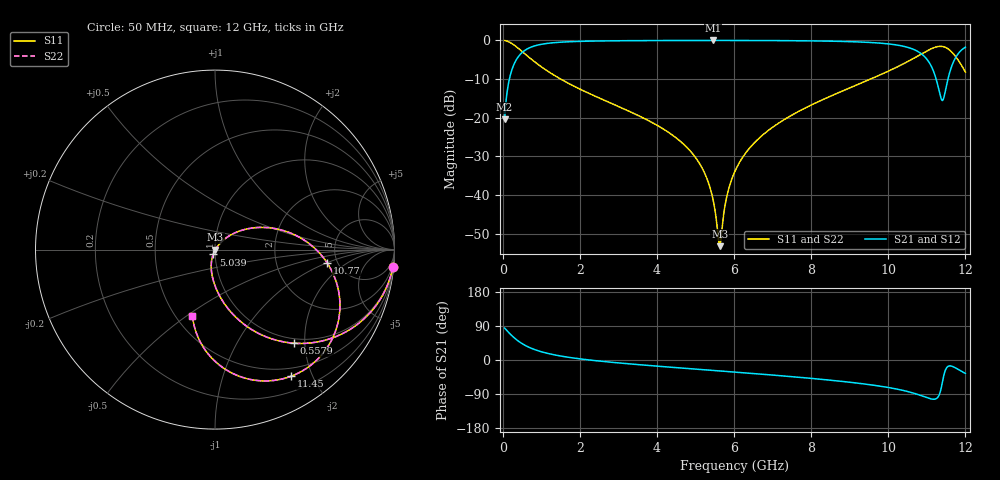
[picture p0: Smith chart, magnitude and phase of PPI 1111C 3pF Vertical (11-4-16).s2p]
# GHz S MA R 50
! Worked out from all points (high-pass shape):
!   1601 points, 50 MHz to 12 GHz, reference 50 ohm
!   highest |S21| = -0.02 dB at 5.457 GHz (marker M1); lowest = -20.4 dB at 50 MHz (marker M2)
!   |S21| within 3 dB of the highest: 518.8 MHz to 10.79 GHz (10.27 GHz wide, 182 % of centre); 11.85 GHz to end of sweep
!   lowest |S11| = -53.3 dB at 5.629 GHz (marker M3), VSWR 1.00, Z = 50.2 - j0.096 ohm
!   |S11| at or under -10 dB: 1.501 GHz to 9.544 GHz (8.043 GHz wide, 146 % of centre)
!   |S22| runs from -53.3 to 0.0 dB; largest |S21 - S12| = 0
!   S11 on the Smith chart (normalised r, x): 50 MHz: 1, -20; 557.9 MHz: 0.91, -1.77; 5.039 GHz: 0.98, -0.05; 10.77 GHz: 4.13, -0.99; 11.45 GHz: 0.39, -1.70; 12 GHz: 0.61, -0.52
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0.05  0.9954 -5.7  0.09534 84.3  0.09534 84.3  0.9954 -5.7
0.2367188  0.9105 -25.7  0.4132 64.3  0.4132 64.3  0.9105 -25.7
0.557875  0.681 -50.0  0.7317 40.0  0.7317 40.0  0.681 -50.0
1.103094  0.4199 -70.9  0.9066 19.0  0.9066 19.0  0.4199 -70.9
2.044156  0.2287 -87.2  0.9722 2.5  0.9722 2.5  0.2287 -87.2
4.038312  0.07778 -105.3  0.9951 -16.5  0.9951 -16.5  0.07778 -105.3
5.039125  0.02863 -110.4  0.9973 -24.3  0.9973 -24.3  0.02863 -110.4
5.293062  0.01646 -109.2  0.9975 -26.3  0.9975 -26.3  0.01646 -109.2
5.457375  0.008605 -103.4  0.9975 -27.6  0.9975 -27.6  0.008605 -103.4
5.584344  0.003013 -73.1  0.9975 -28.5  0.9975 -28.5  0.003013 -73.1
5.629156  0.002168 -26.2  0.9975 -28.9  0.9975 -28.9  0.002168 -26.2
5.823344  0.01006 46.7  0.9974 -30.4  0.9974 -30.4  0.01006 46.7
6.025  0.02026 51.5  0.9971 -31.9  0.9971 -31.9  0.02026 51.5
6.727062  0.05864 49.8  0.9952 -37.5  0.9952 -37.5  0.05864 49.8
8.019156  0.1469 39.8  0.9848 -48.6  0.9848 -48.6  0.1469 39.8
10.01331  0.402 15.0  0.8993 -72.8  0.8993 -72.8  0.402 15.0
10.76766  0.6282 -6.7  0.7177 -91.0  0.7177 -91.0  0.6282 -6.7
11.1635  0.7976 -30.9  0.4101 -103.5  0.4101 -103.5  0.7976 -30.9
11.36516  0.8368 -50.0  0.1794 -77.5  0.1794 -77.5  0.8368 -50.0
11.44731  0.8234 -58.9  0.1863 -37.8  0.1863 -37.8  0.8234 -58.9
11.69378  0.6657 -85.5  0.5316 -18.2  0.5316 -18.2  0.6657 -85.5
12  0.3888 -108.8  0.8164 -35.4  0.8164 -35.4  0.3888 -108.8
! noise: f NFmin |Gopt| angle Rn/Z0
0.05  0.0005244  0.9236  2.687  0.00152
1.372  0.003712  0.6726  8.901  0.002171
2.701  0.005988  0.6161  15.26  0.002854
4.031  0.008095  0.5892  21.57  0.003488
5.36  0.01027  0.5806  27.67  0.004222
6.682  0.01285  0.5901  33.49  0.005293
8.012  0.01674  0.6261  39.21  0.007487
9.341  0.02571  0.7114  45.12  0.01504
10.67  0.07358  0.8781  51.48  0.106
12  0.1107  0.9107  57.43  0.2098
